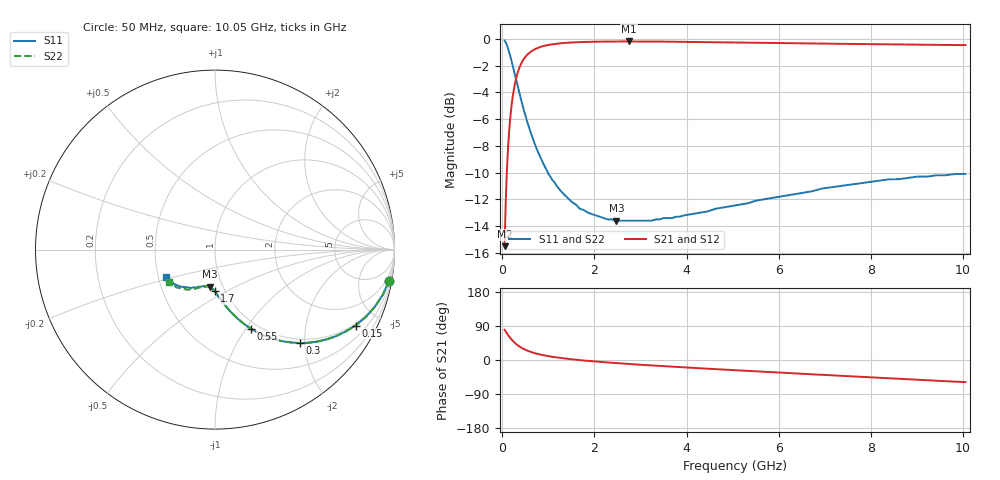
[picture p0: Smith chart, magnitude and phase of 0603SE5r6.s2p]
! AVX Thin Film Operation		Date: August 2001
! Description: Accu-P® Series, Thin Film, SMD, RF Capacitor
! Part Number: 06035J5R6BBT
! 50 MHz  -  10.05 GHz
! Serial Measurements
# mhz S db R 50
!	S11		S21		S12		S22
!	dB	Phase	dB	Phase	dB	Phase	dB	Phase
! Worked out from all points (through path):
!   401 points, 50 MHz to 10.05 GHz, reference 50 ohm
!   highest |S21| = -0.20 dB at 2.75 GHz (marker M1); lowest = -15.5 dB at 50 MHz (marker M2)
!   group delay of S21, straight-line fit = 23.3 ps
!   lowest |S11| = -13.6 dB at 2.475 GHz (marker M3), VSWR 1.53, Z = 43.3 - j18.7 ohm
!   |S11| at or under -10 dB: 988.2 MHz to end of sweep
!   |S22| runs from -13.6 to -0.1 dB; largest |S21 - S12| = 0
!   S11 on the Smith chart (normalised r, x): 50 MHz: 1, -11; 150 MHz: 0.92, -3.74; 300 MHz: 0.92, -1.89; 550 MHz: 0.92, -1.06; 1.7 GHz: 0.89, -0.44; 10.05 GHz: 0.55, -0.19
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50  -0.12 -10.1  -15.50 79.9  -15.50 79.9  -0.12 -10.1
100  -0.48 -19.7  -9.80 70.3  -9.80 70.3  -0.48 -19.7
125  -0.73 -24.2  -8.12 65.8  -8.12 65.8  -0.73 -24.2
150  -1.01 -28.4  -6.83 61.6  -6.83 61.6  -1.01 -28.4
175  -1.32 -32.2  -5.83 57.8  -5.83 57.8  -1.32 -32.2
225  -2.00 -39.1  -4.34 50.8  -4.34 50.8  -2.00 -39.1
300  -3.06 -47.8  -2.96 42.2  -2.96 42.2  -3.06 -47.8
350  -3.78 -52.5  -2.37 37.5  -2.37 37.5  -3.78 -52.5
425  -4.79 -58.3  -1.76 31.7  -1.76 31.7  -4.79 -58.3
550  -6.30 -65.5  -1.16 24.4  -1.16 24.4  -6.30 -65.5
725  -8.04 -72.5  -0.75 17.4  -0.75 17.4  -8.03 -72.5
950  -9.73 -78.7  -0.49 11.3  -0.49 11.3  -9.73 -78.6
1275  -11.39 -84.8  -0.33 5.1  -0.33 5.1  -11.39 -84.7
1700  -12.72 -90.5  -0.25 -0.6  -0.25 -0.6  -12.72 -90.2
1725  -12.75 -90.8  -0.24 -0.8  -0.24 -0.8  -12.75 -90.5
2475  -13.60 -98.3  -0.20 -8.2  -0.20 -8.2  -13.60 -97.6
2750  -13.60 -100.3  -0.20 -10.5  -0.20 -10.5  -13.60 -99.7
3400  -13.50 -105.8  -0.21 -15.5  -0.21 -15.5  -13.50 -104.8
5050  -12.46 -117.8  -0.27 -27.0  -0.27 -27.0  -12.46 -115.4
6725  -11.39 -129.0  -0.35 -37.7  -0.35 -37.7  -11.30 -125.0
8400  -10.50 -140.2  -0.42 -48.2  -0.42 -48.2  -10.49 -135.1
10050  -10.10 -150.8  -0.47 -58.4  -0.47 -58.4  -10.10 -144.8
